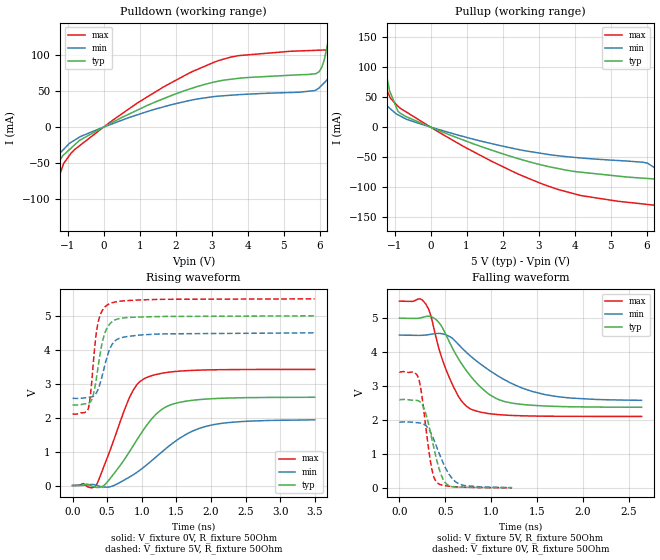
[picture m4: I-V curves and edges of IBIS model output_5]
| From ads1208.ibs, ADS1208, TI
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|   output_5 Model
[Model]   output_5
Model_type   Output
Polarity   Non-Inverting
Vmeas = 2.5
Vref = 2.5
Cref = 30pF
Rref = 50
|   typ   min   max
|   (nom PVT)   (fast PVT)   (slow PVT)
|C_comp from frequency sweep method (F=10MHz)
|C_comp   1.826e-12   1.817e-12   1.882e-12
|ON state : BUFFER OUTPUT TURNED HIGH
|C_comp   1.826e-12   1.817e-12   1.882e-12
|OFF state: BUFFER OUTPUT TURNED LOW
|C_comp   1.633e-12   1.505e-12   1.754e-12
|C_comp from LC tank measurement(L=1nH)
|Resonant Frequency(Hz)   6.330e+09   6.390e+09   5.300e+09
C_comp   6.328e-13   6.210e-13   9.027e-13
|ON state : BUFFER OUTPUT TURNED HIGH
|Resonant Frequency(Hz)   6.330e+09   6.390e+09   5.300e+09
|C_comp   6.328e-13   6.210e-13   9.027e-13
|OFF state: BUFFER OUTPUT TURNED LOW
|Resonant Frequency(Hz)   6.490e+09   6.530e+09   5.390e+09
|C_comp   6.020e-13   5.946e-13   8.728e-13
| Where nom  PVT is Nominal Process, 5V, 35C
|   Fast PVT is Strong Process,  5.5V, -40C
|   Slow PVT is Weak Process,   4.5V, 95C
[Voltage Range]   5   4.5   5.5
|Ambient Temperature   25   85   -40
|Junction Temperature
[Temperature Range]   35   95   -40
[Pullup Reference]   5   4.5   5.5
[Pulldown Reference]   0   0   0
[Power Clamp Reference]   5   4.5   5.5
[GND Clamp Reference]   0   0   0
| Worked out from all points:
|   slope of the pulldown table from 0 to 0.75 V, typ, clamps not added: 39.3 ohm
|   slope of the pullup table from 0 to 0.75 V, typ, clamps not added: 41.7 ohm
|   falling waveform, V_fixture 5V, R_fixture 50Ohm: 20-80 % time 401ps typ, 636ps min, 260ps max; typ from 5 V to 2.38 V
|   rising waveform, V_fixture 0V, R_fixture 50Ohm: 20-80 % time 535ps typ, 749ps min, 382ps max; typ from 0 V to 2.6 V
|   rising waveform, V_fixture 5V, R_fixture 50Ohm: 20-80 % time 141ps typ, 169ps min, 106ps max; typ from 2.37 V to 5 V
|   falling waveform, V_fixture 0V, R_fixture 50Ohm: 20-80 % time 138ps typ, 189ps min, 101ps max; typ from 2.6 V to 0.007 V
[Pulldown]
|   Voltage   I(typ)   I(min)   I(max)
-5V       -394.6mA   -259.2mA   -706.3mA
-2.447V   -158.3mA   -108mA     -267.5mA
-1.375V   -59.3mA    -44.45mA   -87.58mA
-1.111V   -38.58mA   -30.8mA    -50.44mA
-670mV    -18.39mA   -13.85mA   -25.88mA
3.08V     62.55mA    42.34mA    90.1mA
5.9V      74.01mA    51.29mA    106.3mA
6.06V     83.03mA    57.97mA    106.6mA
6.365V    158.5mA    74.94mA    107.2mA
6.891V    386.4mA    105.6mA    110.3mA
7.36V     617.8mA    134.2mA    167.4mA
10V       1.976A     295.4mA    616.1mA
[Pullup]
|   Voltage   I(typ)   I(min)   I(max)
-5V       1.976A     264.8mA    701.6mA
-3.515V   1.206A     173.7mA    447.1mA
-2.095V   484.4mA    87.23mA    205.2mA
-1.56V    226.9mA    55.26mA    115.7mA
-1.375V   145.4mA    44.2mA     84.71mA
-1.14V    60.85mA    31.77mA    51.66mA
-905mV    26.26mA    20.51mA    34.72mA
3.08V     -63.19mA   -43.89mA   -94.42mA
6.021V    -85.73mA   -60.08mA   -129.1mA
6.6V      -90.5mA    -88.32mA   -132.8mA
7.81V     -191.3mA   -159mA     -246.2mA
10V       -395mA     -289.6mA   -620.7mA
[Ramp]
R_load = 50
|   typ   min   max
dV/dt_r   1.56005/5.33975e-10   1.16058/7.48491e-10   2.05282/3.80893e-10
dV/dt_f   1.5755/3.99528e-10   1.15772/6.42155e-10   2.03631/2.6082e-10
[Falling Waveform]
V_fixture = 5V
V_fixture_min = 4.5V
V_fixture_max = 5.5V
R_fixture = 50Ohm
|   Time   V(typ)   V(min)   V(max)
0s        5V         4.5V       5.5V
289ps     5.05V      4.503V     5.41V
343ps     5.047V     4.526V     5.071V
426ps     4.885V     4.551V     4.15V
559ps     4.222V     4.44V      3.158V
675ps     3.67V      4.138V     2.573V
796ps     3.23V      3.836V     2.302V
1.056ns   2.635V     3.33V      2.166V
1.449ns   2.435V     2.842V     2.119V
2.643ns   2.376V     2.58V      2.106V
[Rising Waveform]
V_fixture = 0V
V_fixture_min = 0V
V_fixture_max = 0V
R_fixture = 50Ohm
|   Time   V(typ)   V(min)   V(max)
0s        916pV      1.347nV    889.3pV
342ps     -55.99mV   7.814mV    10.71mV
473ps     38.17mV    -47.76mV   669mV
822ps     996mV      248.9mV    2.593V
930ps     1.346V     389.2mV    2.973V
1.053ns   1.724V     578mV      3.167V
1.206ns   2.1V       841.5mV    3.271V
1.383ns   2.349V     1.146V     3.337V
1.922ns   2.546V     1.741V     3.405V
3.499ns   2.6V       1.934V     3.421V
[Rising Waveform]
V_fixture = 5V
V_fixture_min = 4.5V
V_fixture_max = 5.5V
R_fixture = 50Ohm
|   Time   V(typ)   V(min)   V(max)
0s        2.374V     2.568V     2.106V
227ps     2.418V     2.599V     2.264V
258ps     2.468V     2.605V     2.653V
297ps     2.657V     2.626V     3.546V
363ps     3.411V     2.805V     4.746V
437ps     4.283V     3.306V     5.182V
535ps     4.752V     4.011V     5.357V
646ps     4.903V     4.31V      5.419V
972ps     4.965V     4.434V     5.468V
3.499ns   5V         4.499V     5.5V
[Falling Waveform]
V_fixture = 0V
V_fixture_min = 0V
V_fixture_max = 0V
R_fixture = 50Ohm
|   Time   V(typ)   V(min)   V(max)
0s        2.602V     1.941V     3.422V
155ps     2.581V     1.932V     3.407V
207ps     2.565V     1.92V      3.242V
233ps     2.513V     1.909V     2.927V
275ps     2.295V     1.864V     2.074V
347ps     1.531V     1.596V     648mV
411ps     780.9mV    1.177V     156.5mV
502ps     150.3mV    593.4mV    66.47mV
649ps     25.29mV    121.2mV    28.35mV
1.229ns   7.274mV    11.01mV    4.014mV
